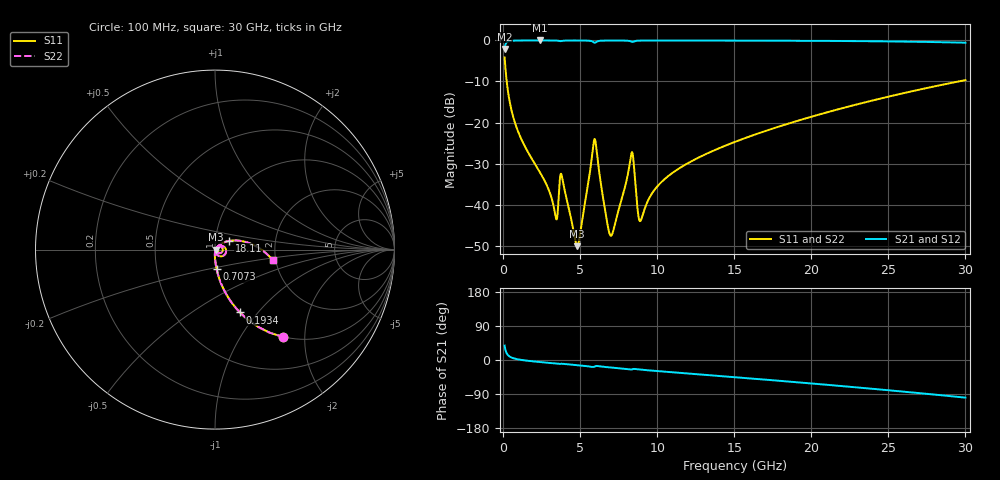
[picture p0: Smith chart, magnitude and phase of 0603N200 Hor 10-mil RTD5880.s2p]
# GHz S MA R 50
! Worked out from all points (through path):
!   3201 points, 100 MHz to 30 GHz, reference 50 ohm
!   highest |S21| = -0.02 dB at 2.38 GHz (marker M1); lowest = -2.1 dB at 100 MHz (marker M2)
!   group delay of S21, straight-line fit = 9.4 ps
!   lowest |S11| = -50.1 dB at 4.809 GHz (marker M3), VSWR 1.01, Z = 50.3 - j0.0942 ohm
!   |S11| at or under -10 dB: 235.9 MHz to 29.56 GHz (29.32 GHz wide, 197 % of centre)
!   |S22| runs from -50.1 to -4.2 dB; largest |S21 - S12| = 0
!   S11 on the Smith chart (normalised r, x): 100 MHz: 0.99, -1.57; 193.4 MHz: 0.99, -0.81; 707.3 MHz: 0.99, -0.22; 18.11 GHz: 1.16, +0.11; 30 GHz: 1.93, -0.26
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0.1  0.6188 -52.0  0.7852 37.9  0.7852 37.9  0.6188 -52.0
0.1934375  0.3768 -68.4  0.9259 21.6  0.9259 21.6  0.3768 -68.4
0.7073438  0.1086 -85.4  0.9933 4.2  0.9933 4.2  0.1086 -85.4
2.379875  0.025 -91.9  0.9982 -5.4  0.9982 -5.4  0.025 -91.9
3.417031  0.007045 -63.7  0.9958 -9.4  0.9958 -9.4  0.007045 -63.7
3.725375  0.02313 -35.1  0.979 -10.1  0.979 -10.1  0.02313 -35.1
3.8375  0.02125 -64.2  0.9874 -9.9  0.9874 -9.9  0.02125 -64.2
4.80925  0.003124 -17.4  0.9968 -13.7  0.9968 -13.7  0.003124 -17.4
5.089563  0.005694 36.1  0.9963 -14.7  0.9963 -14.7  0.005694 36.1
5.9305  0.06275 -8.9  0.9378 -17.4  0.9378 -17.4  0.06275 -8.9
6.734063  0.006377 -59.0  0.995 -18.9  0.995 -18.9  0.006377 -59.0
6.986344  0.004184 -16.6  0.9957 -19.9  0.9957 -19.9  0.004184 -16.6
8.3225  0.04141 12.4  0.9667 -25.0  0.9667 -25.0  0.04141 12.4
8.453312  0.03576 -32.6  0.9646 -23.6  0.9646 -23.6  0.03576 -32.6
8.733625  0.008597 -38.8  0.9915 -24.6  0.9915 -24.6  0.008597 -38.8
8.892469  0.006299 -2.1  0.9941 -25.3  0.9941 -25.3  0.006299 -2.1
10.06978  0.01719 48.8  0.9962 -29.4  0.9962 -29.4  0.01719 48.8
15.05  0.05817 40.7  0.9941 -45.4  0.9941 -45.4  0.05817 40.7
18.10541  0.09185 31.7  0.991 -55.5  0.991 -55.5  0.09185 31.7
20.03956  0.1181 25.6  0.9879 -62.0  0.9879 -62.0  0.1181 25.6
25.01978  0.2068 8.5  0.9721 -79.9  0.9721 -79.9  0.2068 8.5
30  0.3283 -10.5  0.9371 -99.3  0.9371 -99.3  0.3283 -10.5
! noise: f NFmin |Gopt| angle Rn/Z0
0.1  0.0003069  0.9223  0.4336  0.0008737
3.417  0.005531  0.8577  9.744  0.008252
6.743  0.008424  0.8202  19.16  0.009551
10.06  0.008774  0.7539  28.38  0.006774
13.39  0.01041  0.7306  37.43  0.006926
16.7  0.01238  0.7222  46.25  0.00751
20.03  0.01445  0.7189  54.85  0.00807
23.35  0.01661  0.7191  63.16  0.008576
26.67  0.01892  0.722  71.24  0.009032
30  0.02141  0.7271  79.06  0.009441
